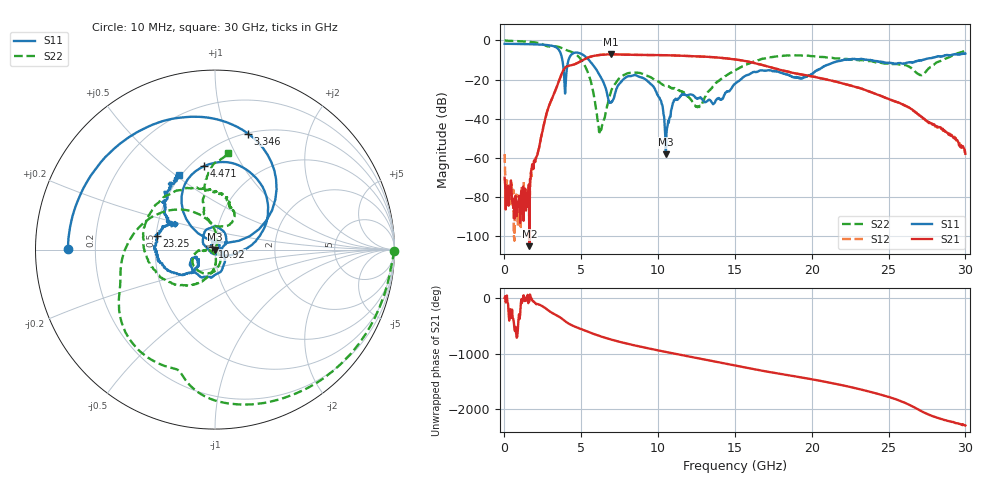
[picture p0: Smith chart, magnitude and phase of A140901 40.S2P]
!  2-Port S-parameters saved by WinCal
! VAR MeasName=S-Parameters (CALIBRATED_DATA) read from VNA (N5244A)
! VAR MeasDate=11/3/2014 9:33:43 AM
! VAR NAME=A140901 40
! VAR FILENAME=A140901 40.S2P
! VAR DATE=11/3/2014 9:33:43 AM
! VAR PHYS_PORTS=1,2
# Hz S RI R 50
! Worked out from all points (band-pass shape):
!   801 points, 10 MHz to 30 GHz, reference 50 ohm
!   highest |S21| = -7.11 dB at 6.908 GHz (marker M1); lowest = -105.1 dB at 1.622 GHz (marker M2)
!   |S21| within 3 dB of the highest: 5.079 GHz to 15.36 GHz (10.28 GHz wide, 101 % of centre)
!   lowest |S11| = -58.1 dB at 10.51 GHz (marker M3), VSWR 1.00, Z = 50.1 - j0.098 ohm
!   |S11| at or under -10 dB: 3.767 GHz to 4.171 GHz (403.6 MHz wide, 10.2 % of centre); 5.498 GHz to 22.06 GHz (16.56 GHz wide, 120 % of centre); 23.83 GHz to 27.23 GHz (3.398 GHz wide, 13.3 % of centre)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
!   |S22| runs from -46.9 to 0.0 dB; largest |S21 - S12| = 0.0025
!   S11 on the Smith chart (normalised r, x): 10 MHz: 0.10, +0.00; 3.346 GHz: 0.51, +1.19; 4.471 GHz: 0.58, +0.70; 10.92 GHz: 0.97, +0.03; 23.25 GHz: 0.50, +0.09; 30 GHz: 0.49, +0.52
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1e7  -0.8175 0.00289  0.000308 4.9e-05  -0.000945 -0.000813  0.9985 -0.00671
3.84875e8  -0.8076 0.1253  -0.000177 4.93e-05  -5.77e-05 -3.95e-05  0.9452 -0.244
1.621962e9  -0.628 0.4965  3.58e-06 -4.27e-06  -1.3e-05 -1.34e-05  0.4562 -0.7991
3.346388e9  0.1837 0.6465  0.0277 0.0496  0.0274 0.0495  -0.4097 -0.5741
3.946188e9  0.00983 0.0429  0.1267 -0.1553  0.1272 -0.1548  -0.5321 -0.2356
4.471012e9  -0.0592 0.4657  -0.1733 -0.1649  -0.1724 -0.1648  -0.485 0.0355
5.033325e9  0.2534 0.3675  -0.2877 0.1025  -0.2879 0.102  -0.2093 0.2229
5.595638e9  0.266 0.104  -0.0634 0.3784  -0.0641 0.3778  0.0036 0.0975
6.232925e9  0.121 -0.0186  0.3428 0.2554  0.3421 0.2559  -0.00599 0.000319
6.9077e9  -0.00956 -0.024  0.4124 -0.1569  0.4124 -0.1563  0.0226 -0.0404
8.4072e9  -0.00527 0.1288  -0.2485 -0.3492  -0.2472 -0.3492  -0.0951 -0.1165
1.001916e10  0.0367 0.00364  -0.3194 0.2772  -0.3198 0.276  -0.0897 -0.00632
1.05065e10  0.000775 -0.000978  -0.1547 0.3903  -0.1552 0.3895  -0.0702 -0.00297
1.091886e10  -0.0144 0.0154  0.00938 0.4137  0.0088 0.4131  -0.0592 -0.00502
1.26058e10  0.0215 0.0247  0.391 -0.0142  0.3907 -0.014  -0.0135 -0.0157
1.5005e10  0.0554 -0.0544  -0.2192 -0.2436  -0.2187 -0.2436  -0.0528 -0.1635
1.71043e10  -0.1151 -0.1282  -0.0966 0.1957  -0.0971 0.1961  -0.3403 -0.1108
2.002832e10  -0.1014 -0.0963  0.1104 -0.0476  0.1116 -0.0477  -0.2395 0.3136
2.325225e10  -0.3243 0.0784  -0.0504 0.0294  -0.0504 0.0299  0.0403 0.3123
2.501416e10  -0.217 0.1482  0.0305 0.00937  0.0305 0.0094  0.0841 0.2437
2.715095e10  -0.2641 0.1716  -0.00516 0.00972  -0.00528 0.00954  0.00643 0.1296
3e10  -0.1979 0.4162  -0.000943 -0.000856  -0.00107 -0.00089  0.0739 0.5366
